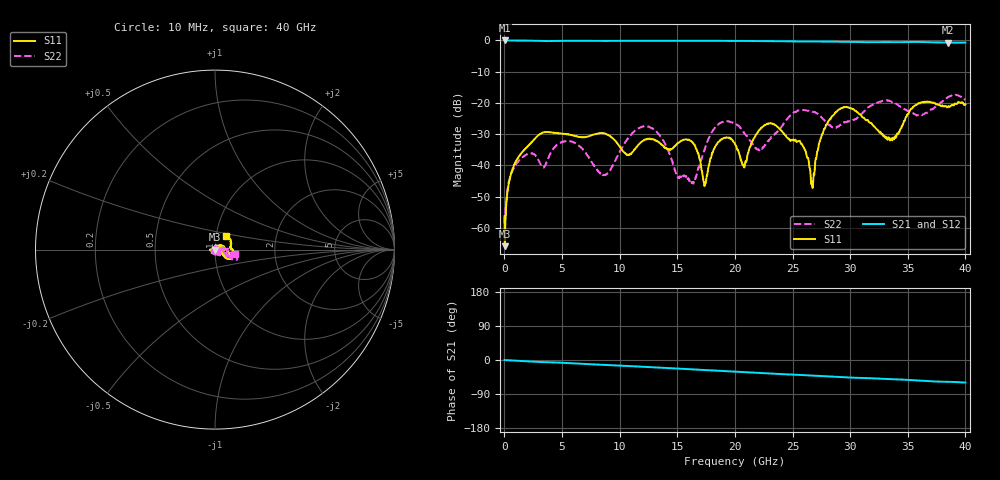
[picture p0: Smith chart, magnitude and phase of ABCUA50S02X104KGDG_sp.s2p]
! Amotech Co.,Ltd.
! http://www.amotech.co.kr/
! Date: Wednesday, December 02, 2020 16:03:11
! Part Number: ABCUA 50S 02X 104K GDG
! Freq. Start=10[MHz] Stop=40[GHz], 4000[Steps]
# Hz S  dB  R 50
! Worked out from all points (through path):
!   4000 points, 10 MHz to 40 GHz, reference 50 ohm
!   highest |S21| = 0.00 dB at 20 MHz (marker M1); lowest = -0.7 dB at 38.52 GHz (marker M2)
!   group delay of S21, straight-line fit = 4.2 ps
!   lowest |S11| = -65.9 dB at 30 MHz (marker M3), VSWR 1.00, Z = 49.9 + j0.00331 ohm
!   |S11| at or under -10 dB: start of sweep to end of sweep
!   |S22| runs from -59.3 to -17.4 dB; largest |S21 - S12| = 0.0035
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1e7  -56.24 -111.3  -0.00 0.1  0.01 0.1  -56.39 -60.0
2e7  -64.61 -136.3  0.00 0.0  0.01 -0.0  -59.32 -22.5
3e7  -65.88 176.3  0.00 -0.0  0.01 -0.0  -59.30 7.5
8.9e8  -39.46 62.9  -0.03 -1.6  -0.02 -1.6  -40.33 80.9
2.72e9  -31.15 26.2  -0.12 -4.8  -0.11 -4.8  -36.95 81.8
6.68e9  -30.98 -50.6  -0.11 -10.1  -0.10 -10.0  -34.42 -85.9
8.7e9  -29.79 -24.2  -0.14 -12.9  -0.13 -12.9  -43.08 -79.6
1.135e10  -34.70 -121.4  -0.10 -16.8  -0.09 -16.8  -28.86 -51.7
1.334e10  -32.47 -126.1  -0.09 -19.9  -0.08 -19.9  -29.77 -53.7
1.625e10  -32.32 -31.6  -0.08 -24.6  -0.07 -24.5  -45.28 -123.9
1.739e10  -45.90 -106.0  -0.10 -26.5  -0.09 -26.4  -34.55 -56.2
1.858e10  -32.46 -176.3  -0.12 -28.5  -0.11 -28.4  -26.79 -48.3
2.001e10  -33.13 -165.7  -0.15 -30.7  -0.14 -30.6  -26.63 -43.0
2.081e10  -40.72 -82.0  -0.15 -32.0  -0.14 -31.9  -29.77 -27.7
2.336e10  -26.78 3.3  -0.23 -36.1  -0.21 -36.0  -30.35 11.3
2.579e10  -33.08 83.1  -0.32 -39.7  -0.30 -39.6  -22.24 -23.6
2.667e10  -45.26 55.5  -0.34 -41.0  -0.33 -40.9  -22.75 -28.5
2.915e10  -21.89 -25.1  -0.42 -44.9  -0.40 -44.8  -27.01 14.3
3.334e10  -31.02 28.4  -0.53 -50.3  -0.52 -50.2  -19.29 -29.2
3.581e10  -20.51 -33.4  -0.48 -54.0  -0.47 -53.8  -23.98 -4.1
3.852e10  -21.08 9.0  -0.70 -57.6  -0.69 -57.4  -18.14 -24.4
4e10  -20.47 51.9  -0.67 -59.5  -0.66 -59.4  -19.06 -13.4
